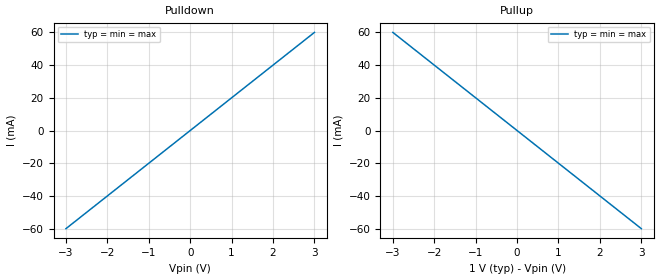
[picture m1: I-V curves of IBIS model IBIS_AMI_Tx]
|Copyright 2009 Signal Integrity Software, Inc.
|  Signal Integrity Software, Inc. (SiSoft)
[IBIS Ver] 5.0
[Disclaimer]
Permission to use, copy, modify, and distribute this software and
associated documentation for educational, research and commercial
purposes, without fee and without a signed licensing agreement, is hereby
granted, provided that the above copyright notice, this paragraph and
the following three paragraphs appear in all copies, modifications, and
distributions.
This is part of a sample IBIS Algorithmic Modeling Interface (AMI) model.
This code has been provided by SiSoft to help demonstrate and drive
adoption of the IBIS AMI modeling standard.  For more information
on this and other IBIS AMI models, contact Signal Integrity Software,
6 Clock Tower Place, Maynard, MA 01754, (978) 461-0449 or email
ibis-ami@sisoft.com.
THIS MATERIAL IS PROVIDED FOR THE RECIPIENT'S USE AT THE RECIPIENT's OWN RISK.
IN NO EVENT SHALL SISOFT BE LIABLE TO ANY PARTY FOR FOR ANY DIRECT,
INDIRECT, INCIDENTAL,SPECIAL OR CONSEQUENTIAL DAMAGES, OR ANY OTHER DAMAGES
WHATSOEVER (INCLUDING, WITHOUT LIMITATION, DAMAGES FOR LOSS OF BUSINESS PROFITS,
BUSINESS INTERRUPTION, LOSS OF BUSINESS INFORMATION, OR OTHER PECUNIARY LOSS)
ARISING OUT OF THE USE OR INABILITY TO USE THIS LICENSED MATERIAL, WHETHER
OR NOT THE POSSIBILITY OR CAUSE OF SUCH DAMAGES WAS KNOWN TO SISOFT.
SISOFT SPECIFICALLY DISCLAIMS ANY WARRANTIES, INCLUDING, BUT NOT
LIMITED TO, THE IMPLIED WARRANTIES OF MERCHANTABILITY AND FITNESS FOR A
PARTICULAR PURPOSE. THIS SOFTWARE AND ACCOMPANYING DOCUMENTATION, IF
ANY, PROVIDED HEREUNDER IS PROVIDED "AS IS". SISOFT HAS NO OBLIGATION
TO PROVIDE MAINTENANCE, SUPPORT, UPDATES, ENHANCEMENTS, OR
MODIFICATIONS.
[File Name]  sisoft_tx.ibs
[File Rev]   1.0
[Date]   8/25/2009
[Source]   Developed by: Signal Integrity Software, Inc.
6 Clock Tower Place, Suite 250 Maynard, MA 01754
[Notes]
Rev 1.0
- 8/25/2009 Inital Release
[Copyright]   Copyright 2009, Signal Integrity Software, Inc.
[Component] SiSoft_Tx
[Manufacturer] SiSoft
[Package]
R_pkg 0.001m   NA   NA
L_pkg 0.001nH  NA   NA
C_pkg 0.001pF  NA   NA
[Pin]   signal_name   model_name   R_pin L_pin  C_pin
1p   SiSoft_AMI_Tx   IBIS_AMI_Tx
1n   SiSoft_AMI_Tx_L   IBIS_AMI_Tx
[Diff_Pin] inv_pin vdiff tdelay_typ tdelay_min tdelay_max
1p   1n   0.1V  NA   NA   NA
| Models and submodels in the file (1): IBIS_AMI_Tx (Output)
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[Model] IBIS_AMI_Tx
Model_type Output
C_comp 0.5p 0.45p 0.55p
Cref = 0
Vref = 0.5
Rref = 50
Vmeas = 0.5
[Temperature_Range] 25 100 0
[Voltage Range] 1.0 0.9 1.1
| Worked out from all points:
|   slope of the pulldown table from 0 to 0.15 V, typ, clamps not added: 50 ohm
|   slope of the pullup table from 0 to 0.15 V, typ, clamps not added: 50 ohm
[Pulldown]
-3V       -60mA      -60mA      -60mA
0V        0A         0A         0A
3V        60mA       60mA       60mA
[Pullup]
-3V       60mA       60mA       60mA
0V        0A         0A         0A
3V        -60mA      -60mA      -60mA
[GND Clamp]
-3V       0A         0A         0A
0V        0A         0A         0A
3V        0A         0A         0A
[Power Clamp]
-3V       0A         0A         0A
0V        0A         0A         0A
3V        0A         0A         0A
[Ramp]
dV/dt_r .45/50p .42/55p .48/45p
dV/dt_f .45/50p .42/55p .48/45p
[Algorithmic Model]
Executable Windows_VisualStudio_32 IBIS_AMI_Tx.dll IBIS_AMI_Tx.ami
Executable linux_gcc3.2.3_32 libIBIS_AMI_Tx.so IBIS_AMI_Tx.ami
[End Algorithmic Model]
